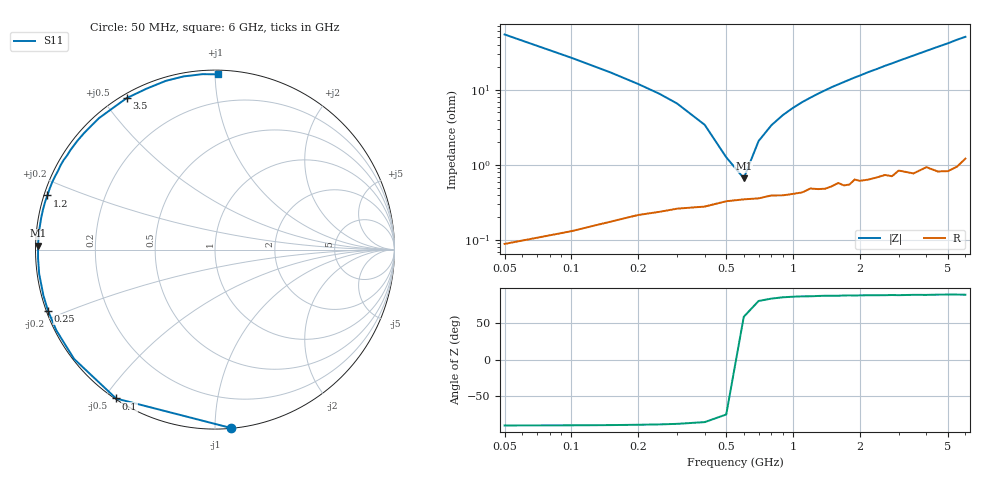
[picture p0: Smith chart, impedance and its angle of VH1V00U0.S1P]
! Infineon Technologies  Discrete & RF Semiconductors
! BB 814
! Si Tuning Diode in SOT23
! VR = 1 V
! S-Parameters:  July  1999
# GHz  S  MA  R  50
!  f  S11
! GHz  MAG  ANG
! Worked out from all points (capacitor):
!   34 points, 50 MHz to 6 GHz, reference 50 ohm
!   read as one part to ground: C = 57.7 pF near 50 MHz
!   lowest |Z| = 665 mohm at 600 MHz (marker M1)
!   series resonance near 568.3 MHz, so ESL is about 1.4 nH
!   S11 on the Smith chart (normalised r, x): 50 MHz: 0.00, -1.10; 100 MHz: 0.00, -0.54; 250 MHz: 0.00, -0.18; 1.2 GHz: 0.01, +0.16; 3.5 GHz: 0.02, +0.57; 6 GHz: 0.02, +1.02
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0.05  0.9984 -84.8
0.1  0.9959 -123.6
0.15  0.9938 -142.2
0.2  0.9919 -153.0
0.25  0.9908 -159.9
0.3  0.9898 -165.0
0.4  0.989 -172.2
0.5  0.987 -177.2
0.6  0.9862 178.7
0.7  0.9858 175.3
0.8  0.9845 172.3
1  0.9839 166.9
1.1  0.9832 164.4
1.2  0.9812 162.1
1.4  0.9816 157.6
1.6  0.9785 153.4
1.8  0.9798 149.4
2.2  0.9774 141.7
2.4  0.9764 138.3
2.6  0.9753 134.6
2.8  0.9768 131.4
3  0.9732 128.0
3.5  0.9771 120.3
4  0.9744 113.0
4.5  0.9792 106.3
5  0.9807 100.3
5.5  0.9799 94.0
6  0.9765 88.9
